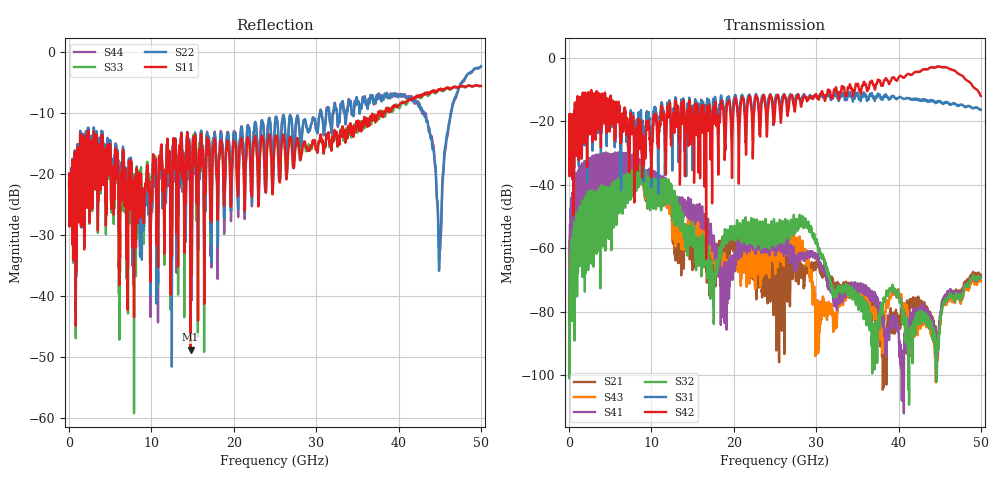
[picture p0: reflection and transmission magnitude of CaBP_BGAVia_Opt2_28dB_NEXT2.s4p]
!* Samtec Inc. NovaRay Examax Flyover System  *
!*  REV DATE  = 08/08/18  *
!*  TYPE  = TOUCHSTONE  *
!*  PORTS  = 4 port  *
!*  UNITS  = GHz  *
!*  DATA RANGE = DC  to 50 GHz; 10 MHz Step  *
!*  PARAMETER  = S  *
!*  FORMAT  = Real-Imaginary  *
!*  REFERENCE  = 50 ohms  *
!*  SOURCE  = HFSS  *
!*  VALIDATED  = No  *
!*  MANUFACTURER = SAMTEC  *
!*  INTERCONNECT = NVAx to EBCx to EBCx to NVAx  *
!*  [Full Channel NVAx to EBCx to EBCx to NVAx  with PCB Trace and BGA Via]  *
!*  BOUNDARY A  = Silicon BGA Ball Pad  *
!*  BOUNDARY B  = Silicon BGA Ball Pad  *
!*  NVAx (end a) ->>- (end b) NVAx  *
!*  Port 01 ->>- Port 02  *
!*  Port 03 ->>- Port 04  *
!***************************** CHANNEL MODEL ******************************************
# GHz S RI R 50
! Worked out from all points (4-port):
!   5000 points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, 10 MHz to 50 GHz, reference 50 ohm
!   strongest paths, dB at 10 MHz, 12.51 GHz, 25.01 GHz, 37.51 GHz, 50 GHz:
!     S42: -23.1, -20.8, -16.3, -6.8, -12.0
!     S31: -23.1, -28.5, -13.0, -11.3, -16.4
!     S32: -85.4, -44.2, -59.1, -84.8, -69.4
!     S41: -72.0, -48.6, -60.6, -76.1, -69.3
!     S43: -75.7, -52.0, -67.3, -88.3, -70.3
!     S21: -76.8, -52.4, -67.9, -79.5, -68.5
!   lowest |S11| = -48.8 dB at 14.75 GHz (marker M1), VSWR 1.01, Z = 49.7 - j0.221 ohm
!   |S11| at or under -10 dB: start of sweep to 37.51 GHz; 37.83997 GHz to 38.00552 GHz (165.6 MHz wide, 0.437 % of centre); 38.04261 GHz to 38.22467 GHz (182.1 MHz wide, 0.477 % of centre)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
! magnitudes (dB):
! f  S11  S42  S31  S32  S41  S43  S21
! 10 MHz  -22.1  -23.1  -23.1  -85.4  -72.0  -75.7  -76.8
! 6.13 GHz  -29.1  -17.5  -19.3  -37.6  -29.8  -33.1  -33.3
! 14.75 GHz  -48.8  -21.9  -22.0  -55.6  -47.0  -51.6  -56.1
! 18.57 GHz  -15.9  -15.3  -13.7  -58.5  -66.7  -63.9  -60.5
! 40.41 GHz  -8.3  -5.9  -12.6  -80.0  -108.0  -77.5  -79.5
! 44.99 GHz  -6.2  -2.7  -13.9  -86.0  -83.6  -84.5  -84.8
! 50 GHz  -5.6  -12.0  -16.4  -69.4  -69.3  -70.3  -68.5
